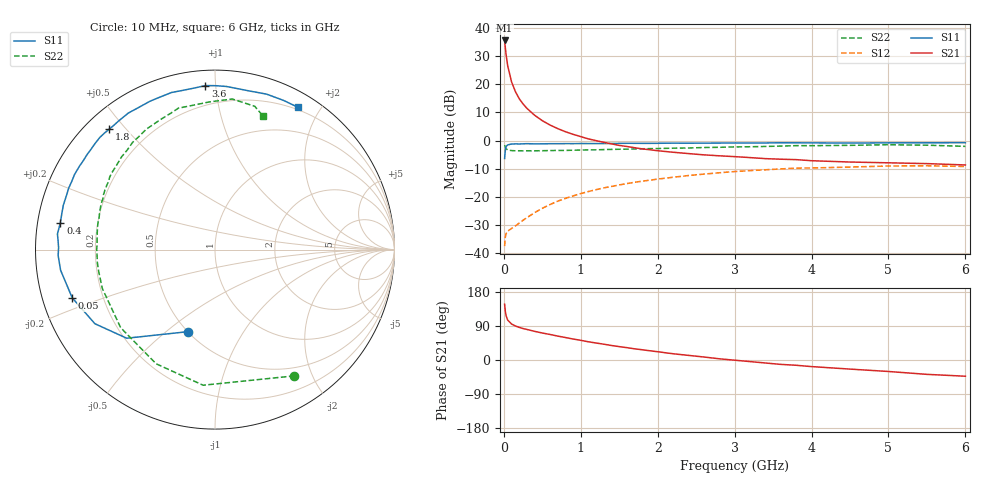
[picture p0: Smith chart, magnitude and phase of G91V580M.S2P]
! SIEMENS Small Signal Semiconductors
! BFG235
! Si NPN RF Bipolar Junction Transistor in SOT223
! VCE = 1.5 V  IC = 80 mA
! Common Emitter S-Parameters:  July  1994
# GHz  S  MA  R  50
!  f  S11  S21  S12  S22
! GHz  MAG  ANG  MAG  ANG  MAG  ANG  MAG  ANG
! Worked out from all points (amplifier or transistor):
!   40 points, 10 MHz to 6 GHz, reference 50 ohm
!   highest |S21| = 35.6 dB at 10 MHz (marker M1)
!   |S21| within 3 dB of that: start of sweep to 21.17 MHz
!   unconditionally stable (mu >= 1): 448.6 MHz to 1.655 GHz; 1.731 GHz to 1.917 GHz
!   at 200 MHz: K = 0.77, MSG = 22.1 dB, |S12| = -29.3 dB
!   at 1.5 GHz: K = 1.02, MAG = 6.2 dB, |S12| = -15.8 dB
!   at 6 GHz: K = 0.95, MSG = 0.3 dB, |S12| = -9.2 dB
!   S11 on the Smith chart (normalised r, x): 10 MHz: 0.50, -0.60; 50 MHz: 0.09, -0.16; 400 MHz: 0.07, +0.09; 1.8 GHz: 0.07, +0.45; 3.6 GHz: 0.08, +0.94; 6 GHz: 0.17, +1.73
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0.01  0.4812 -108.2  60.21 147.1  0.0133 58.6  0.8312 -57.8
0.02  0.697 -134.9  44.05 127.4  0.0196 42.1  0.7586 -95.0
0.03  0.7862 -148.3  33.21 116.1  0.0223 34.5  0.7157 -117.3
0.05  0.8396 -161.3  21.42 105.3  0.0245 28.2  0.6822 -140.4
0.1  0.8679 -172.4  11.11 95.0  0.0275 31.4  0.6642 -161.0
0.15  0.8745 -177.8  7.44 89.7  0.0304 37.8  0.6593 -169.3
0.2  0.8716 179.2  5.558 86.1  0.0342 42.2  0.6595 -173.9
0.25  0.8762 176.5  4.478 83.0  0.0384 46.5  0.6577 -177.1
0.3  0.8822 174.3  3.743 80.6  0.0427 49.9  0.659 -179.9
0.4  0.8743 170.1  2.823 75.6  0.0524 53.5  0.6584 176.2
0.5  0.8767 166.8  2.26 71.2  0.0626 55.6  0.6617 173.1
0.6  0.8805 163.7  1.891 67.4  0.0731 56.5  0.6649 170.1
0.7  0.8808 160.0  1.635 63.1  0.0838 56.6  0.6687 167.4
0.9  0.8838 154.7  1.293 55.4  0.104 55.0  0.6742 162.6
1.1  0.8867 148.3  1.072 48.0  0.1245 52.7  0.6841 157.9
1.8  0.8929 131.2  0.712 27.0  0.19 41.1  0.7168 143.2
2.2  0.9011 122.4  0.621 16.5  0.2233 33.7  0.7335 135.2
3.2  0.9051 101.4  0.499 -4.2  0.2927 14.3  0.7776 116.2
3.6  0.9155 93.4  0.467 -11.6  0.3138 6.0  0.799 107.9
4.5  0.9042 78.3  0.416 -24.0  0.3387 -9.6  0.8235 92.1
5.5  0.9147 65.3  0.39 -37.9  0.3569 -27.2  0.8286 74.5
6  0.9178 59.8  0.369 -42.8  0.3465 -33.8  0.7895 70.0
